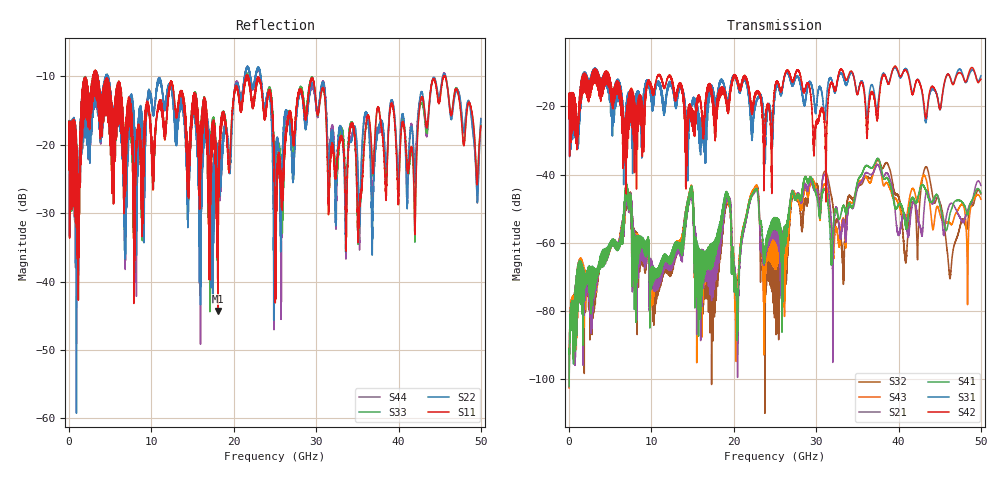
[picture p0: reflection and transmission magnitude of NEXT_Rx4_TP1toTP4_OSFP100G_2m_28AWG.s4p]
! Touchstone data
! Created: 27-Feb-2019 by IdEM 12 (12.1.0)
! COMMENTS
!  Created Wed Feb 27 12:03:36 2019
!  64 Port Network Data from SP1.SP block
!  freq  magS1_1  angS1_1  magS1_2  angS1_2  magS1_3  angS1_3  magS1_4  angS1_4
!  magS1_5  angS1_5  magS1_6  angS1_6  magS1_7  angS1_7  magS1_8  angS1_8
!  magS1_9  angS1_9  magS1_10  angS1_10  magS1_11  angS1_11  magS1_12  angS1_12
!  magS1_13  angS1_13  magS1_14  angS1_14  magS1_15  angS1_15  magS1_16  angS1_16
!  magS1_17  angS1_17  magS1_18  angS1_18  magS1_19  angS1_19  magS1_20  angS1_20
!  magS1_21  angS1_21  magS1_22  angS1_22  magS1_23  angS1_23  magS1_24  angS1_24
!  magS1_25  angS1_25  magS1_26  angS1_26  magS1_27  angS1_27  magS1_28  angS1_28
!  magS1_29  angS1_29  magS1_30  angS1_30  magS1_31  angS1_31  magS1_32  angS1_32
!  magS1_33  angS1_33  magS1_34  angS1_34  magS1_35  angS1_35  magS1_36  angS1_36
!  magS1_37  angS1_37  magS1_38  angS1_38  magS1_39  angS1_39  magS1_40  angS1_40
!  magS1_41  angS1_41  magS1_42  angS1_42  magS1_43  angS1_43  magS1_44  angS1_44
!  magS1_45  angS1_45  magS1_46  angS1_46  magS1_47  angS1_47  magS1_48  angS1_48
!  magS1_49  angS1_49  magS1_50  angS1_50  magS1_51  angS1_51  magS1_52  angS1_52
!  magS1_53  angS1_53  magS1_54  angS1_54  magS1_55  angS1_55  magS1_56  angS1_56
!  magS1_57  angS1_57  magS1_58  angS1_58  magS1_59  angS1_59  magS1_60  angS1_60
!  magS1_61  angS1_61  magS1_62  angS1_62  magS1_63  angS1_63  magS1_64  angS1_64
!  magS2_1  angS2_1  magS2_2  angS2_2  magS2_3  angS2_3  magS2_4  angS2_4
!  magS2_5  angS2_5  magS2_6  angS2_6  magS2_7  angS2_7  magS2_8  angS2_8
!  magS2_9  angS2_9  magS2_10  angS2_10  magS2_11  angS2_11  magS2_12  angS2_12
!  magS2_13  angS2_13  magS2_14  angS2_14  magS2_15  angS2_15  magS2_16  angS2_16
!  magS2_17  angS2_17  magS2_18  angS2_18  magS2_19  angS2_19  magS2_20  angS2_20
!  magS2_21  angS2_21  magS2_22  angS2_22  magS2_23  angS2_23  magS2_24  angS2_24
!  magS2_25  angS2_25  magS2_26  angS2_26  magS2_27  angS2_27  magS2_28  angS2_28
!  magS2_29  angS2_29  magS2_30  angS2_30  magS2_31  angS2_31  magS2_32  angS2_32
!  magS2_33  angS2_33  magS2_34  angS2_34  magS2_35  angS2_35  magS2_36  angS2_36
!  magS2_37  angS2_37  magS2_38  angS2_38  magS2_39  angS2_39  magS2_40  angS2_40
!  magS2_41  angS2_41  magS2_42  angS2_42  magS2_43  angS2_43  magS2_44  angS2_44
!  magS2_45  angS2_45  magS2_46  angS2_46  magS2_47  angS2_47  magS2_48  angS2_48
!  magS2_49  angS2_49  magS2_50  angS2_50  magS2_51  angS2_51  magS2_52  angS2_52
!  magS2_53  angS2_53  magS2_54  angS2_54  magS2_55  angS2_55  magS2_56  angS2_56
!  magS2_57  angS2_57  magS2_58  angS2_58  magS2_59  angS2_59  magS2_60  angS2_60
!  magS2_61  angS2_61  magS2_62  angS2_62  magS2_63  angS2_63  magS2_64  angS2_64
!  magS3_1  angS3_1  magS3_2  angS3_2  magS3_3  angS3_3  magS3_4  angS3_4
!  magS3_5  angS3_5  magS3_6  angS3_6  magS3_7  angS3_7  magS3_8  angS3_8
!  magS3_9  angS3_9  magS3_10  angS3_10  magS3_11  angS3_11  magS3_12  angS3_12
!  magS3_13  angS3_13  magS3_14  angS3_14  magS3_15  angS3_15  magS3_16  angS3_16
!  magS3_17  angS3_17  magS3_18  angS3_18  magS3_19  angS3_19  magS3_20  angS3_20
!  magS3_21  angS3_21  magS3_22  angS3_22  magS3_23  angS3_23  magS3_24  angS3_24
!  magS3_25  angS3_25  magS3_26  angS3_26  magS3_27  angS3_27  magS3_28  angS3_28
!  magS3_29  angS3_29  magS3_30  angS3_30  magS3_31  angS3_31  magS3_32  angS3_32
!  magS3_33  angS3_33  magS3_34  angS3_34  magS3_35  angS3_35  magS3_36  angS3_36
!  magS3_37  angS3_37  magS3_38  angS3_38  magS3_39  angS3_39  magS3_40  angS3_40
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# Hz S MA R 50
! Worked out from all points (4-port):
!   5000 points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, 10 MHz to 50 GHz, reference 50 ohm
!   strongest paths, dB at 10 MHz, 12.51 GHz, 25.01 GHz, 37.51 GHz, 50 GHz:
!     S42: -18.0, -12.6, -14.0, -21.6, -12.0
!     S31: -18.0, -14.0, -15.8, -18.9, -11.0
!     S41: -102.2, -65.5, -53.0, -35.3, -45.3
!     S21: -102.0, -67.5, -55.7, -37.2, -43.2
!     S43: -102.6, -66.8, -58.2, -35.4, -47.2
!     S32: -101.5, -69.0, -62.9, -35.5, -45.7
!   lowest |S11| = -44.3 dB at 18.09 GHz (marker M1), VSWR 1.01, Z = 49.5 + j0.362 ohm
!   |S11| at or under -10 dB: 3.49 GHz to 21.47 GHz (17.98 GHz wide, 144 % of centre); 21.77 GHz to 45.47 GHz (23.7 GHz wide, 70.5 % of centre); 45.66 GHz to end of sweep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
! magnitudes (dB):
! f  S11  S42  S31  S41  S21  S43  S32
! 10 MHz  -17.7  -18.0  -18.0  -102.2  -102.0  -102.6  -101.5
! 7.16 GHz  -16.4  -29.0  -19.3  -47.3  -48.5  -47.0  -48.2
! 10.01 GHz  -20.0  -15.0  -18.8  -67.2  -65.0  -68.5  -66.6
! 14.77 GHz  -16.8  -23.4  -21.2  -44.2  -45.1  -44.3  -45.3
! 18.09 GHz  -44.3  -20.0  -16.7  -57.0  -58.8  -58.0  -60.2
! 46.26 GHz  -14.9  -11.5  -11.4  -51.3  -48.6  -54.2  -70.1
! 50 GHz  -17.2  -12.0  -11.0  -45.3  -43.2  -47.2  -45.7
